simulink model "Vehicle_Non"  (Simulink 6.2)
settings: Solver=ode3  StartTime=0.0  StopTime=1000  FixedStep=Ts  RelTol=1e-3
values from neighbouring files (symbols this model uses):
  ini = [wbo; atto; Hco]    [start.m]    (also in start1.m; start2.m; start3.m)
  nt = 12    [start.m]    (also in start1.m; start2.m; start3.m)
undefined symbols (not defined in the file or in its folder): Rigbod_Dynam_LVLH

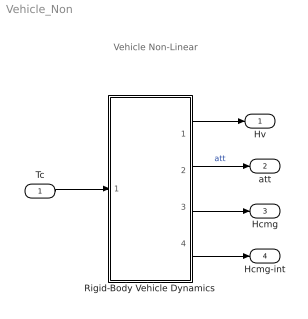
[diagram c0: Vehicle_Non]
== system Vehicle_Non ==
  note: Vehicle Non-Linear
  Tc : Inport  Port=1  PortDimensions=3  LatchInput=off
  Rigid-Body Vehicle Dynamics : Subsystem
  Hv : Outport
  att : Outport  Port=2
  Hcmg : Outport  Port=3
  Hcmg-int : Outport  Port=4
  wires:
  Rigid-Body Vehicle Dynamics/3(Hcmg) -> Hcmg/1
  Rigid-Body Vehicle Dynamics/4(Hint) -> Hcmg-int/1
  Rigid-Body Vehicle Dynamics/1(wb) -> Hv/1
  Rigid-Body Vehicle Dynamics/2(atti-lv) -> att/1  "att"
  Tc/1 -> Rigid-Body Vehicle Dynamics/1(Tc)

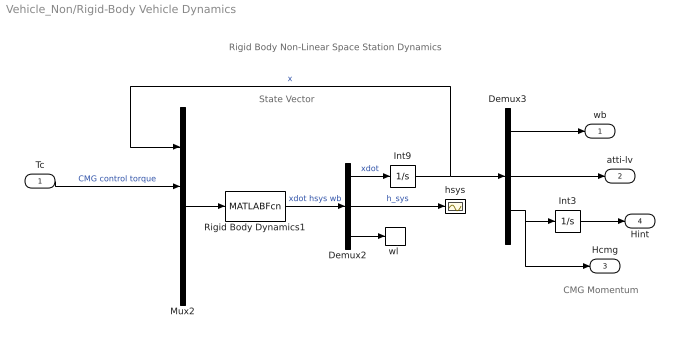
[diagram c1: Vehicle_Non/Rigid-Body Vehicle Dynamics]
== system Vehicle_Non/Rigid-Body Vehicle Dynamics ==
  note: Rigid Body Non-Linear Space Station Dynamics
  note: State Vector
  note: CMG Momentum
  Tc : Inport  Port=1  PortDimensions=3  LatchInput=off
  Demux2 : Demux  Outputs=[9,3,3]
  Demux3 : Demux  Outputs=[3,3,3]
  Int3 : Integrator
  Int9 : Integrator  InitialCondition=ini
  Mux2 : Mux  Inputs=[9, 3, 3, nt]
  Rigid Body Dynamics1 : MATLABFcn  MATLABFcn=Rigbod_Dynam_LVLH( u(1:9), u(10:12), u(13:15), u(16:15+nt) )  OutputDimensions=15
  hsys : Scope
  "wl " : ToWorkspace  VariableName=wl  SampleTime=-1  SaveFormat=Array
  wb : Outport
  atti-lv : Outport  Port=2
  Hcmg : Outport  Port=3
  Hint : Outport  Port=4
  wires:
  Rigid Body Dynamics1/1 -> Demux2/1  "xdot hsys wb"
  Demux2/1 -> Int9/1  "xdot"
  Int9/1 -> Demux3/1, Mux2/1  "x"
  Tc/1 -> Mux2/2  "CMG control torque"
  Demux2/3 -> "wl "/1
  Demux2/2 -> hsys/1  "h_sys"
  Demux3/1 -> wb/1
  Demux3/2 -> atti-lv/1
  Demux3/3 -> Int3/1, Hcmg/1
  Int3/1 -> Hint/1
  Mux2/1 -> Rigid Body Dynamics1/1
